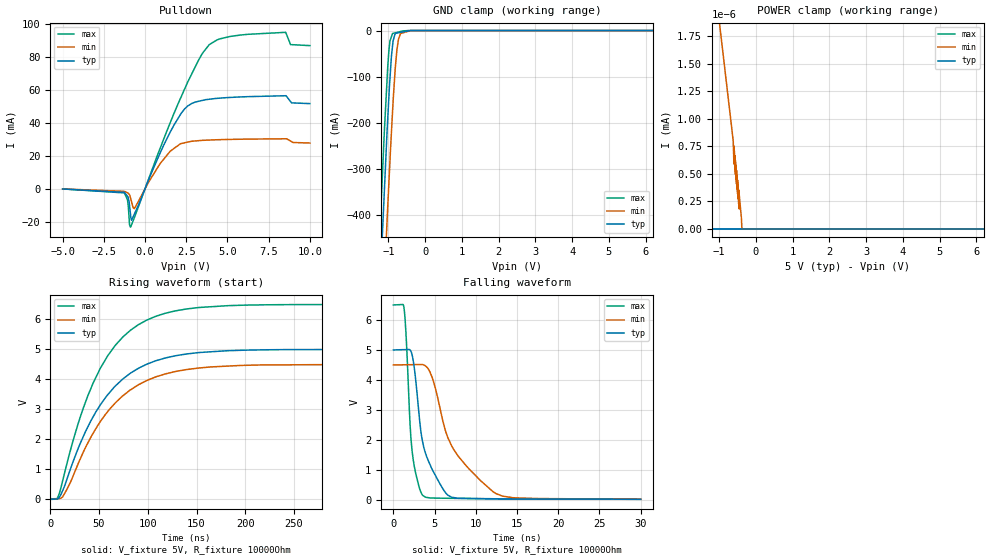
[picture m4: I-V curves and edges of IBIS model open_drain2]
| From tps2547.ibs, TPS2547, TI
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|   open_drain2 Model
[Model]   open_drain2
Model_type   Open_drain
Polarity   Non-Inverting
Vmeas = 2.5
Vref = 5
Cref = 10pF
Rref = 10000
|   typ   min   max
C_comp   0.6392pF   0.5366pF   0.7441pF
|  Where Nom  PVT is Nominal Process,   5V,  27C
|   Fast PVT is Strong Process,   6.5V, -40C
|   Slow PVT is Weak Process,   4.5V, 125C
[Voltage Range]   5   4.5   6.5
|Junction Temperature
[Temperature Range]   27   125   -40
[Pullup Reference]   5   4.5   6.5
[Pulldown Reference]   0   -0   0
[Power Clamp Reference]   5   4.5   6.5
[GND Clamp Reference]   0   0   0
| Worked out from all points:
|   slope of the pulldown table from 0 to 0.75 V, typ, clamps not added: 41.9 ohm
|   GND clamp passes 1 mA (typ) near -0.46 V on its own axis
|   POWER clamp passes 1 mA (typ) near -3.63 V on its own axis
|   falling waveform, V_fixture 5V, R_fixture 10000Ohm: 20-80 % time 2ns typ, 4.39ns min, 827ps max; typ from 5 V to 0.02 V
|   rising waveform, V_fixture 5V, R_fixture 10000Ohm: 20-80 % time 53.2ns typ, 55.1ns min, 50.5ns max; typ from 0.02 V to 5 V
[Pulldown]
|   Voltage   I(typ)   I(min)   I(max)
-5V       -165.7uA   -152.3uA   -146.3uA
-1.25V    -2.253mA   -1.616mA   -2.561mA
-1.065V   -4.618mA   -2.485mA   -6.743mA
-940.2mV  -10.28mA   -3.763mA   -21.94mA
-883.5mV  -15.62mA   -5.59mA    -23.36mA
-644.4mV  -15.34mA   -12.01mA   -17.46mA
942.9mV   22.29mA    15.59mA    25.22mA
2.178V    45.55mA    27.38mA    55.48mA
3.892V    54.3mA     29.53mA    87.42mA
8.535V    56.43mA    30.3mA     94.92mA
8.827V    52.89mA    28.93mA    87.47mA
10V       51.65mA    27.72mA    86.85mA
[GND Clamp]
|   Voltage   I(typ)   I(min)   I(max)
-5V       -7.959A    -8.136A    -7.854A
-1.25V    -593.6mA   -795.1mA   -467.8mA
-1.108V   -344.8mA   -541.4mA   -216mA
-1.036V   -218.4mA   -412.5mA   -106.6mA
-986.3mV  -144.1mA   -330.6mA   -43.98mA
-958.1mV  -105.2mA   -284.6mA   -22.8mA
-886.7mV  -33.46mA   -176.1mA   -6.524mA
-814.6mV  -7.314mA   -83.35mA   -5.061mA
-768mV    -5.476mA   -41.56mA   -4.114mA
-722.5mV  -4.816mA   -17.86mA   -3.192mA
-393mV    -33.71uA   -187.7uA   -24.73uA
10V       0A         0A         0A
[POWER Clamp]
|   Voltage   I(typ)   I(min)   I(max)
-5V       223.5mA    118.7mA    505.5mA
-2.067V   8.818uA    4.49uA     236.6uA
-1.25V    0A         3.236nA    7.132nA
-1.25V    0A         3.101nA    0A
-1.036V   0A         2nA        0A
-821.5mV  0A         1.386nA    0A
-467.7mV  0A         227.2pA    0A
-467.5mV  0A         354.5pA    0A
-452.8mV  0A         182pA      0A
-452.7mV  0A         309.8pA    0A
-380.7mV  0A         0A         0A
10V       0A         0A         0A
[Ramp]
R_load = 10000
|   typ   min   max
dV/dt_r   2.98809/5.33052e-08   2.68546/5.51757e-08   3.88595/5.04783e-08
dV/dt_f   2.98809/2.00317e-09   2.68546/4.37265e-09   3.88595/8.26894e-10
[Falling Waveform]
V_fixture = 5V
V_fixture_min = 4.5V
V_fixture_max = 6.5V
R_fixture = 10000Ohm
C_fixture = 0F
|   Time   V(typ)   V(min)   V(max)
0s        5V         4.5V       6.5V
1.277ns   5.01V      4.505V     6.421V
1.518ns   5.012V     4.506V     5.598V
2.001ns   5.003V     4.508V     2.635V
2.231ns   4.877V     4.509V     1.741V
3.561ns   1.921V     4.51V      151.8mV
4.712ns   1.014V     4.079V     62.35mV
6.613ns   158.2mV    2.075V     54.85mV
12.28ns   38.43mV    240.2mV    32.53mV
30ns      19.84mV    24.01mV    23.42mV
[Rising Waveform]
V_fixture = 5V
V_fixture_min = 4.5V
V_fixture_max = 6.5V
R_fixture = 10000Ohm
C_fixture = 0F
|   Time   V(typ)   V(min)   V(max)
0s        19.84mV    24.01mV    23.42mV
8.527ns   33.67mV    20.06mV    123.6mV
16.49ns   611.7mV    294.3mV    1.114V
30.74ns   1.863V     1.345V     2.743V
51.3ns    3.147V     2.59V      4.37V
74.44ns   4.014V     3.452V     5.416V
98.63ns   4.502V     3.957V     5.974V
127.9ns   4.786V     4.26V      6.285V
182.3ns   4.958V     4.445V     6.462V
400ns     5V         4.5V       6.5V
